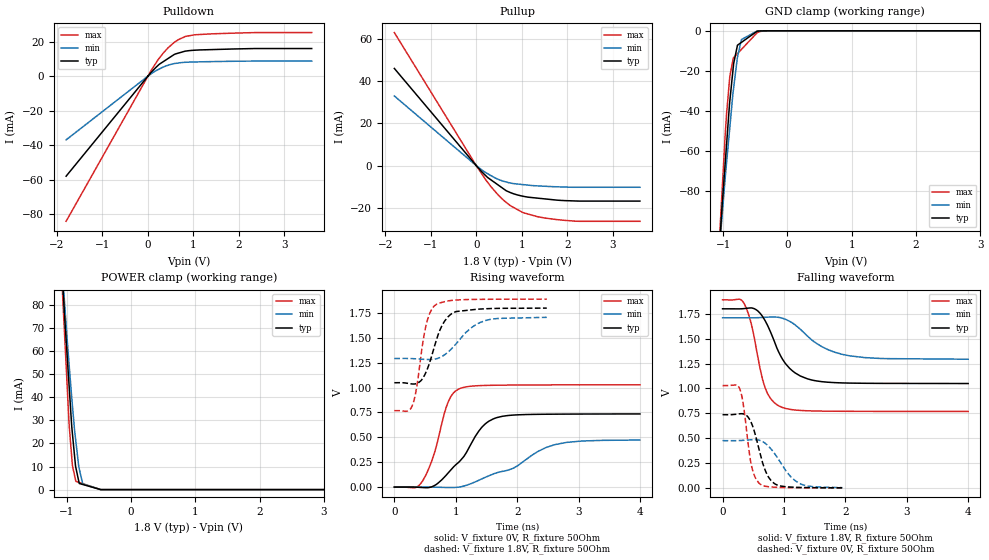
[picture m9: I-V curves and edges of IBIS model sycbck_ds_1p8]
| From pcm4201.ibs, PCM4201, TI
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|   sycbck_ds_1p8 Model
[Model]   sycbck_ds_1p8
Model_type   I/O
Polarity   Non-Inverting
Enable   Active-Low
Vinl = 0.54
Vinh = 1.26
Vmeas = 0.9
Vref = 0.9
Cref = 2pF
Rref = 50
|   typ   min   max
|   (nom PVT)   (fast PVT)   (slow PVT)
|C_comp from frequency sweep method (F=6.94MHz)
|Average
C_comp   1.424e-12   1.242e-12   1.621e-12
|ON state : BUFFER OUTPUT TURNED HIGH
|C_comp   1.510e-12   1.305e-12   1.739e-12
|OFF state: BUFFER IN HIGH IMPEDANCE
|C_comp   1.338e-12   1.179e-12   1.504e-12
|C_comp from LC tank measurement(L=1nH)
|Average
|Resonant Frequency(Hz)   7.410e+09   7.675e+09   7.155e+09
|C_comp   4.618e-13   4.304e-13   4.953e-13
|ON state : BUFFER OUTPUT TURNED HIGH
|Resonant Frequency(Hz)   7.400e+09   7.640e+09   7.170e+09
|C_comp   4.630e-13   4.344e-13   4.932e-13
|OFF state: BUFFER IN HIGH IMPEDANCE
|Resonant Frequency(Hz)   7.420e+09   7.710e+09   7.140e+09
|C_comp   4.605e-13   4.265e-13   4.974e-13
| Where nom  PVT is Nominal Process, 1.8V, 35C
|   Fast PVT is Strong Process,  1.89V, -10C
|   Slow PVT is Weak Process,   1.71V, 80C
[Model Spec]
Vinl   0.54   0.513   0.567
Vinh   1.26   1.197   1.323
[Voltage Range]   1.8   1.71   1.89
|Ambient Temperature   25   70   -10
|Junction Temperature
[Temperature Range]   35   80   -10
[Pullup Reference]   1.8   1.71   1.89
[Pulldown Reference]   0   0   0
[Power Clamp Reference]   1.8   1.71   1.89
[GND Clamp Reference]   0   0   0
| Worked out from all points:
|   slope of the pulldown table from 0 to 0.27 V, typ, clamps not added: 37.4 ohm
|   slope of the pullup table from 0 to 0.27 V, typ, clamps not added: 45.3 ohm
|   GND clamp passes 1 mA (typ) near -0.51 V on its own axis
|   falling waveform, V_fixture 1.8V, R_fixture 50Ohm: 20-80 % time 377ps typ, 566ps min, 242ps max; typ from 1.8 V to 1.05 V
|   rising waveform, V_fixture 0V, R_fixture 50Ohm: 20-80 % time 524ps typ, 937ps min, 283ps max; typ from 0 V to 0.736 V
|   rising waveform, V_fixture 1.8V, R_fixture 50Ohm: 20-80 % time 255ps typ, 400ps min, 172ps max; typ from 1.05 V to 1.8 V
|   falling waveform, V_fixture 0V, R_fixture 50Ohm: 20-80 % time 208ps typ, 333ps min, 136ps max; typ from 0.736 V to 0.001 V
[Pulldown]
|   Voltage   I(typ)   I(min)   I(max)
-1.8V     -57.89mA   -36.89mA   -83.98mA
75.6mV    2.32mA     1.436mA    3.522mA
226.8mV   6.318mA    3.809mA    9.639mA
332.6mV   8.293mA    5.198mA    13.23mA
440.4mV   10.15mA    6.265mA    16.32mA
574.6mV   12.46mA    7.222mA    19.42mA
663.4mV   13.26mA    7.557mA    21.02mA
825.9mV   14.46mA    7.994mA    22.96mA
1.058V    15.03mA    8.196mA    23.95mA
2.366V    15.95mA    8.681mA    25.18mA
3.6V      15.95mA    8.681mA    25.18mA
[GND Clamp]
|   Voltage   I(typ)   I(min)   I(max)
-1.8V     -506.3mA   -422.2mA   -629.4mA
-1.051V   -104.7mA   -105.9mA   -99.82mA
-1.015V   -86.71mA   -91.79mA   -79.1mA
-969.6mV  -66.65mA   -73.72mA   -52.58mA
-950.7mV  -58.34mA   -67.11mA   -43.19mA
-895.9mV  -34.76mA   -47.95mA   -22.49mA
-837mV    -16.38mA   -28.49mA   -13.39mA
-777.6mV  -7.171mA   -13.18mA   -11.37mA
-716.5mV  -5.777mA   -4.369mA   -9.286mA
-470.6mV  -190uA     -45.19uA   -906.7uA
-357.2mV  -9.976uA   -3.626uA   -60.98uA
3.6V      0A         0A         0A
[Pullup]
|   Voltage   I(typ)   I(min)   I(max)
-1.8V     46.08mA    33mA       63.1mA
20.08fV   -9.81pA    -7.712pA   -13.6pA
213.6mV   -4.889mA   -3.416mA   -6.898mA
485.7mV   -9.281mA   -6.558mA   -14mA
657mV     -11.91mA   -7.795mA   -17.47mA
752.2mV   -12.84mA   -8.313mA   -19.06mA
1.058V    -14.7mA    -9.111mA   -22.54mA
1.382V    -15.55mA   -9.689mA   -24.41mA
1.784V    -16.44mA   -10.09mA   -25.67mA
2.268V    -16.87mA   -10.31mA   -26.46mA
3.6V      -16.87mA   -10.31mA   -26.46mA
[POWER Clamp]
|   Voltage   I(typ)   I(min)   I(max)
-1.8V     485.5mA    403.7mA    605.4mA
-1.062V   89.95mA    92.35mA    83.52mA
-1.033V   75.38mA    80.96mA    67.43mA
-963.9mV  45.55mA    54.71mA    28.98mA
-923.4mV  28.12mA    40.32mA    14.72mA
-911mV    24.26mA    36.39mA    10.47mA
-862.2mV  10.1mA     22.02mA    4.108mA
-812.3mV  3.643mA    9.925mA    3.148mA
-804.6mV  2.654mA    9.001mA    3.077mA
-750.7mV  2.225mA    2.486mA    2.582mA
-470.3mV  3.961uA    2.627uA    8.482uA
3.6V      0A         0A         0A
[Ramp]
R_load = 50
|   typ   min   max
dV/dt_r   0.441368/5.23045e-10   0.283939/9.31949e-10   0.616949/2.82498e-10
dV/dt_f   0.450474/3.76601e-10   0.249915/5.60403e-10   0.672853/2.41317e-10
[Falling Waveform]
V_fixture = 1.8V
V_fixture_min = 1.71V
V_fixture_max = 1.89V
R_fixture = 50Ohm
|   Time   V(typ)   V(min)   V(max)
0s        1.8V       1.71V      1.89V
356ps     1.802V     1.71V      1.847V
470ps     1.809V     1.71V      1.641V
688ps     1.686V     1.714V     1.015V
792ps     1.551V     1.717V     889.9mV
938ps     1.336V     1.711V     817.7mV
1.272ns   1.123V     1.591V     778.5mV
1.606ns   1.069V     1.423V     772.1mV
1.954ns   1.055V     1.341V     770.3mV
3.998ns   1.049V     1.293V     768.6mV
[Rising Waveform]
V_fixture = 0V
V_fixture_min = 0V
V_fixture_max = 0V
R_fixture = 50Ohm
|   Time   V(typ)   V(min)   V(max)
0s        642.3pV    1.279nV    373.2pV
340ps     -448uV     319.3uV    -5.828mV
456ps     -4.46mV    254.4uV    57.89mV
658ps     17.07mV    -1.036mV   354mV
872ps     139.3mV    -4.061mV   848.9mV
1.056ns   254.6mV    532uV      988.2mV
1.428ns   604.1mV    83.67mV    1.021V
1.674ns   699.5mV    145.1mV    1.024V
2.612ns   733.2mV    426.6mV    1.028V
3.998ns   735.6mV    473.2mV    1.028V
[Rising Waveform]
V_fixture = 1.8V
V_fixture_min = 1.71V
V_fixture_max = 1.89V
R_fixture = 50Ohm
|   Time   V(typ)   V(min)   V(max)
0s        1.049V     1.293V     768.5mV
216ps     1.043V     1.293V     764.6mV
298ps     1.037V     1.292V     828.7mV
360ps     1.04V      1.289V     990.9mV
518ps     1.159V     1.283V     1.632V
654ps     1.417V     1.286V     1.823V
814ps     1.664V     1.329V     1.864V
994ps     1.763V     1.432V     1.88V
1.49ns    1.793V     1.676V     1.888V
2.482ns   1.8V       1.707V     1.89V
[Falling Waveform]
V_fixture = 0V
V_fixture_min = 0V
V_fixture_max = 0V
R_fixture = 50Ohm
|   Time   V(typ)   V(min)   V(max)
0s        736.1mV    475.1mV    1.028V
282ps     745.1mV    476.4mV    992.3mV
340ps     743.7mV    478.5mV    828mV
466ps     657.4mV    484.2mV    237.2mV
592ps     391.6mV    479.7mV    49.01mV
726ps     133.3mV    431.9mV    13.7mV
888ps     29.41mV    309mV      5.97mV
1.078ns   9.612mV    135.3mV    3.127mV
1.248ns   5.172mV    46.84mV    2.13mV
1.948ns   1.366mV    3.323mV    776.5uV
